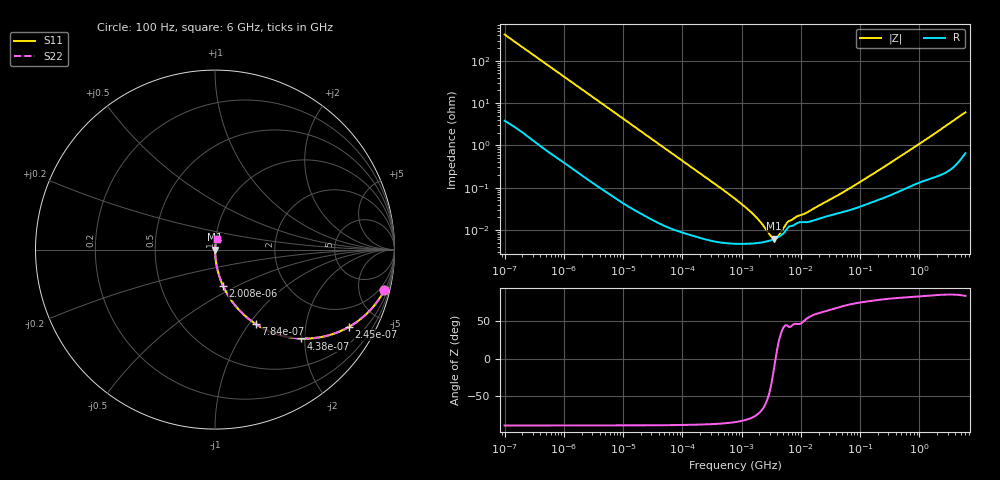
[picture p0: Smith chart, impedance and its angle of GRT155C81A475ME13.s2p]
!Murata Part Number: GRT155C81A475ME13
!These Parameters are Measured in Series Mode Connection
!Data Generated on Jun 19, 2026
!  o--ll--o
!Port1  Port2
!  o------o
!Operation Temp=25[degC], DC Bias Voltage=0[V]
!Freq. Start=100[Hz] Stop=6[GHz] 401[Steps]
# Hz S RI R 50
!Freq.(Hz) S11(Real) S11(Imag) S21(Real) S21(Imag) S12(Real) S12(Imag) S22(Real) S22(Imag)
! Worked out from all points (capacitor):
!   401 points, 100 Hz to 6 GHz, reference 50 ohm
!   read as one part in series: C = 3.8 uF near 109 Hz
!   lowest |Z| = 6.24 mohm at 3.55 MHz (marker M1)
!   series resonance near 3.753 MHz, so ESL is about 470 pH
!   S11 on the Smith chart (normalised r, x): 100 Hz: 1.08, -8.35; 245 Hz: 1.03, -3.43; 438 Hz: 1.02, -1.93; 784 Hz: 1.01, -1.08; 2.008 kHz: 1.00, -0.42; 6 GHz: 1.01, +0.12
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100  0.944 -0.2255  0.056 0.2255  0.056 0.2255  0.944 -0.2255
164  0.8654 -0.3365  0.1346 0.3365  0.1346 0.3365  0.8654 -0.3365
245  0.7447 -0.4313  0.2553 0.4313  0.2553 0.4313  0.7447 -0.4313
335  0.6116 -0.4828  0.3884 0.4828  0.3884 0.4828  0.6116 -0.4828
438  0.4812 -0.4951  0.5188 0.4951  0.5188 0.4951  0.4812 -0.4951
784  0.2276 -0.4147  0.7724 0.4147  0.7724 0.4147  0.2276 -0.4147
1227  0.109 -0.3071  0.891 0.3071  0.891 0.3071  0.109 -0.3071
2008  0.0447 -0.202  0.9553 0.202  0.9553 0.202  0.0447 -0.202
3437  0.0163 -0.122  0.9837 0.122  0.9837 0.122  0.0163 -0.122
6433  0.00505 -0.0662  0.995 0.0662  0.995 0.0662  0.00505 -0.0662
40335  0.000259 -0.0107  0.9997 0.0107  0.9997 0.0107  0.000259 -0.0107
774597  4.75e-05 -0.000544  1 0.000544  1 0.000544  4.75e-05 -0.000544
1516199  4.79e-05 -0.000243  1 0.000243  1 0.000243  4.79e-05 -0.000243
2594782  5.33e-05 -8.84e-05  0.9999 8.84e-05  0.9999 8.84e-05  5.33e-05 -8.84e-05
2837864  5.5e-05 -6.63e-05  0.9999 6.63e-05  0.9999 6.63e-05  5.5e-05 -6.63e-05
3549919  6.1e-05 -1.3e-05  0.9999 1.3e-05  0.9999 1.3e-05  6.1e-05 -1.3e-05
4643984  7.47e-05 5.07e-05  0.9999 -5.07e-05  0.9999 -5.07e-05  7.47e-05 5.07e-05
6353432  0.000121 0.00011  0.9999 -0.00011  0.9999 -0.00011  0.000121 0.00011
1.555665e7  0.000164 0.000258  0.9998 -0.000258  0.9998 -0.000258  0.000164 0.000258
5.960426e7  0.000281 0.00083  0.9997 -0.00083  0.9997 -0.00083  0.000281 0.00083
3.124326e8  0.00066 0.00368  0.9993 -0.00368  0.9993 -0.00368  0.00066 0.00368
6e9  0.00997 0.0589  0.99 -0.0589  0.99 -0.0589  0.00997 0.0589
